(* Logix 5000 AddOnInstructionDefinition export AMCI_3601_AOP_Program_Blend_Move; software revision 20.03 *)

ADD_ON_INSTRUCTION AMCI_3601_AOP_Program_Blend_Move   (* revision 0.0 *)
// Revision note:
// 3/2020: Version 0 is the initial release
VAR_INPUT
   Status_Bits_MSW : INT; {required}
   Status_Bits_LSW : INT; {required}
        .9   // The 3601 module sets this bit to Acknowledge the receipt of a blend move programming block
   Number_of_Segments : INT; {required}
   Final_Move_Deceleration : INT; {required}
   Acceleration_Type_segments_9_to_16 : INT;
   Acceleration_Type_segments_1_to_8 : INT;
   Segment_1_Distance : DINT; {required}
   Segment_1_Programmed_Speed : DINT; {required}
   Segment_1_Acceleration_Deceleration : INT; {required}
   Segment_2_Distance : DINT; {required}
   Segment_2_Programmed_Speed : DINT; {required}
   Segment_2_Acceleration_Deceleration : INT; {required}
   Segment_3_Distance : DINT; {required}
   Segment_3_Programmed_Speed : DINT; {required}
   Segment_3_Acceleration_Deceleration : INT; {required}
   Segment_4_Distance : DINT; {required}
   Segment_4_Programmed_Speed : DINT; {required}
   Segment_4_Acceleration_Deceleration : INT; {required}
   Segment_5_Distance : DINT; {required}
   Segment_5_Programmed_Speed : DINT; {required}
   Segment_5_Acceleration_Deceleration : INT; {required}
   Segment_6_Distance : DINT; {required}
   Segment_6_Programmed_Speed : DINT; {required}
   Segment_6_Acceleration_Deceleration : INT; {required}
   Segment_7_Distance : DINT; {required}
   Segment_7_Programmed_Speed : DINT; {required}
   Segment_7_Acceleration_Deceleration : INT; {required}
   Segment_8_Distance : DINT; {required}
   Segment_8_Programmed_Speed : DINT; {required}
   Segment_8_Acceleration_Deceleration : INT; {required}
   Segment_9_Distance : DINT; {required}
   Segment_9_Programmed_Speed : DINT; {required}
   Segment_9_Acceleration_Deceleration : INT; {required}
   Segment_10_Distance : DINT; {required}
   Segment_10_Programmed_Speed : DINT; {required}
   Segment_10_Acceleration_Deceleration : INT; {required}
   Segment_11_Distance : DINT; {required}
   Segment_11_Programmed_Speed : DINT; {required}
   Segment_11_Acceleration_Deceleration : INT; {required}
   Segment_12_Distance : DINT; {required}
   Segment_12_Programmed_Speed : DINT; {required}
   Segment_12_Acceleration_Deceleration : INT; {required}
   Segment_13_Distance : DINT; {required}
   Segment_13_Programmed_Speed : DINT; {required}
   Segment_13_Acceleration_Deceleration : INT; {required}
   Segment_14_Distance : DINT; {required}
   Segment_14_Programmed_Speed : DINT; {required}
   Segment_14_Acceleration_Deceleration : INT; {required}
   Segment_15_Distance : DINT; {required}
   Segment_15_Programmed_Speed : DINT; {required}
   Segment_15_Acceleration_Deceleration : INT; {required}
   Segment_16_Distance : DINT; {required}
   Segment_16_Programmed_Speed : DINT; {required}
   Segment_16_Acceleration_Deceleration : INT; {required}
END_VAR
VAR_OUTPUT
   Blend_Move_Programmed : BOOL; {access Read Only, visible}
END_VAR
VAR_IN_OUT
   AMCI_3601_output_data : AM:1769_3601:O:0; {required}
END_VAR
VAR
   command_data_block : INT[8];
   Blend_Move_setup : INT[8] := ([1] := 768);
   Blend_Move_counter : COUNTER;
   Programmed_Speed : DINT;
   Distance : DINT;
   upper_result_X_1000 : DINT;
END_VAR

ROUTINE Logic   (* ladder *)
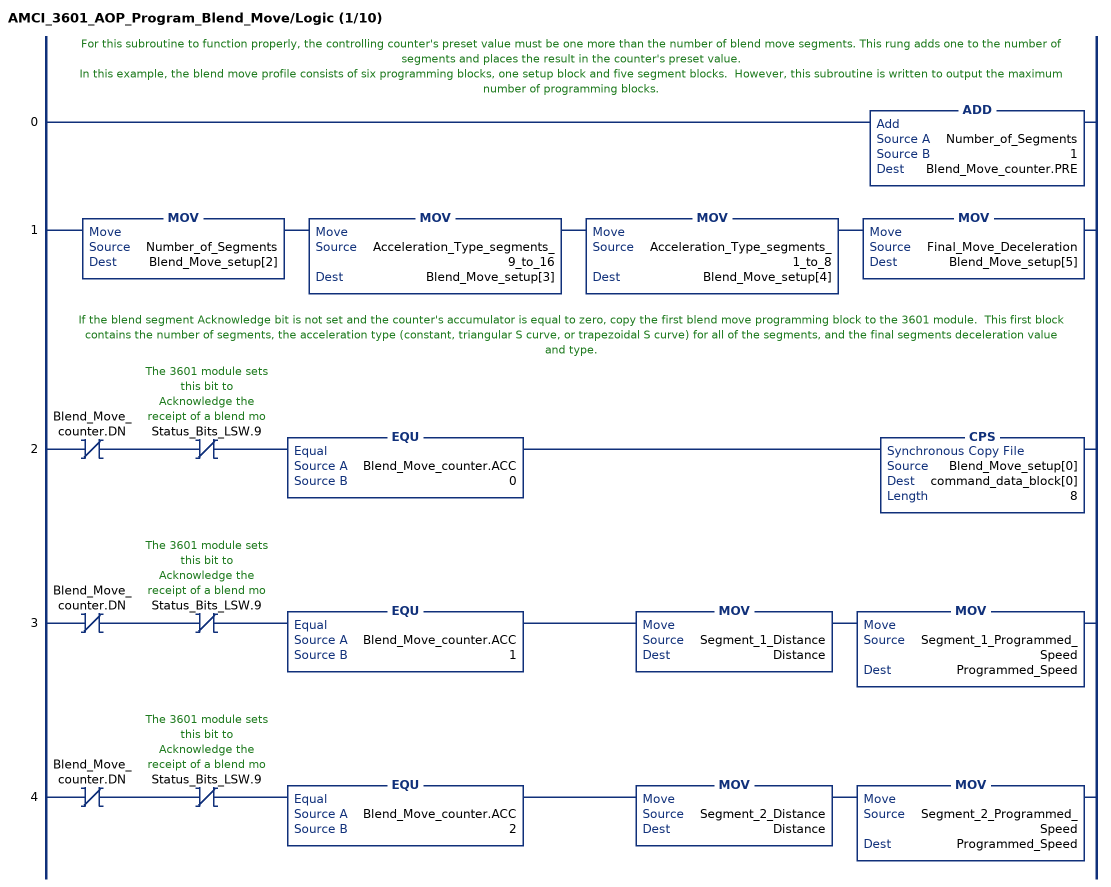
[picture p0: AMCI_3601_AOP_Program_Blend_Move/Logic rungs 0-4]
   // For this subroutine to function properly, the controlling counter's preset value must be one more than the number of blend move segments. This rung adds one to the number of segments and places the result in the counter's preset value.
   // In this example, the blend move profile consists of six programming blocks, one setup block and five segment blocks.  However, this subroutine is written to output the maximum number of programming blocks.
   0: ADD(Number_of_Segments,1,Blend_Move_counter.PRE);
   1: MOV(Number_of_Segments,Blend_Move_setup[2])MOV(Acceleration_Type_segments_9_to_16,Blend_Move_setup[3])MOV(Acceleration_Type_segments_1_to_8,Blend_Move_setup[4])MOV(Final_Move_Deceleration,Blend_Move_setup[5]);
   // If the blend segment Acknowledge bit is not set and the counter's accumulator is equal to zero, copy the first blend move programming block to the 3601 module.  This first block contains the number of segments, the acceleration type (constant, triangular S curve, or trapezoidal S curve) for all of the segments, and the final segments deceleration value and type.
   2: XIO(Blend_Move_counter.DN)XIO(Status_Bits_LSW.9)EQU(Blend_Move_counter.ACC,0)CPS(Blend_Move_setup[0],command_data_block[0],8);
   3: XIO(Blend_Move_counter.DN)XIO(Status_Bits_LSW.9)EQU(Blend_Move_counter.ACC,1)MOV(Segment_1_Distance,Distance)MOV(Segment_1_Programmed_Speed,Programmed_Speed);
   4: XIO(Blend_Move_counter.DN)XIO(Status_Bits_LSW.9)EQU(Blend_Move_counter.ACC,2)MOV(Segment_2_Distance,Distance)MOV(Segment_2_Programmed_Speed,Programmed_Speed);
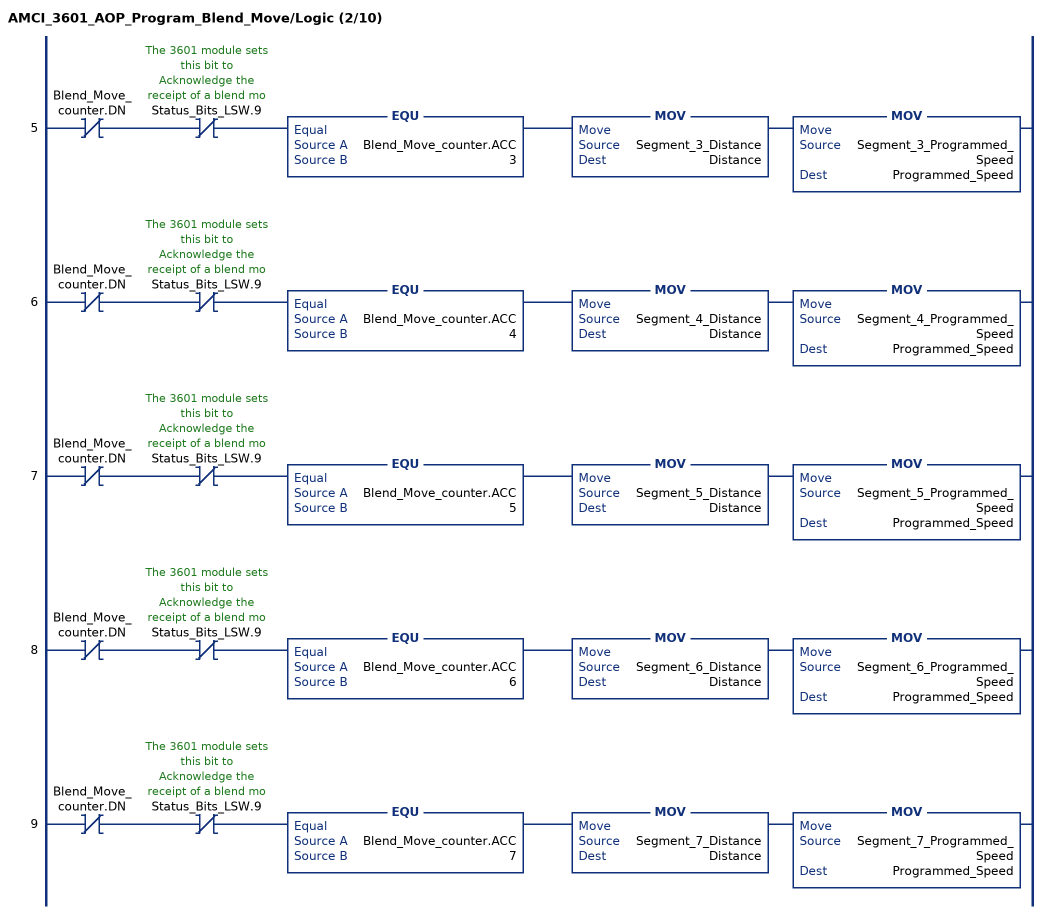
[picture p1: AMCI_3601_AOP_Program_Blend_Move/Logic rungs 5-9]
   5: XIO(Blend_Move_counter.DN)XIO(Status_Bits_LSW.9)EQU(Blend_Move_counter.ACC,3)MOV(Segment_3_Distance,Distance)MOV(Segment_3_Programmed_Speed,Programmed_Speed);
   6: XIO(Blend_Move_counter.DN)XIO(Status_Bits_LSW.9)EQU(Blend_Move_counter.ACC,4)MOV(Segment_4_Distance,Distance)MOV(Segment_4_Programmed_Speed,Programmed_Speed);
   7: XIO(Blend_Move_counter.DN)XIO(Status_Bits_LSW.9)EQU(Blend_Move_counter.ACC,5)MOV(Segment_5_Distance,Distance)MOV(Segment_5_Programmed_Speed,Programmed_Speed);
   8: XIO(Blend_Move_counter.DN)XIO(Status_Bits_LSW.9)EQU(Blend_Move_counter.ACC,6)MOV(Segment_6_Distance,Distance)MOV(Segment_6_Programmed_Speed,Programmed_Speed);
   9: XIO(Blend_Move_counter.DN)XIO(Status_Bits_LSW.9)EQU(Blend_Move_counter.ACC,7)MOV(Segment_7_Distance,Distance)MOV(Segment_7_Programmed_Speed,Programmed_Speed);
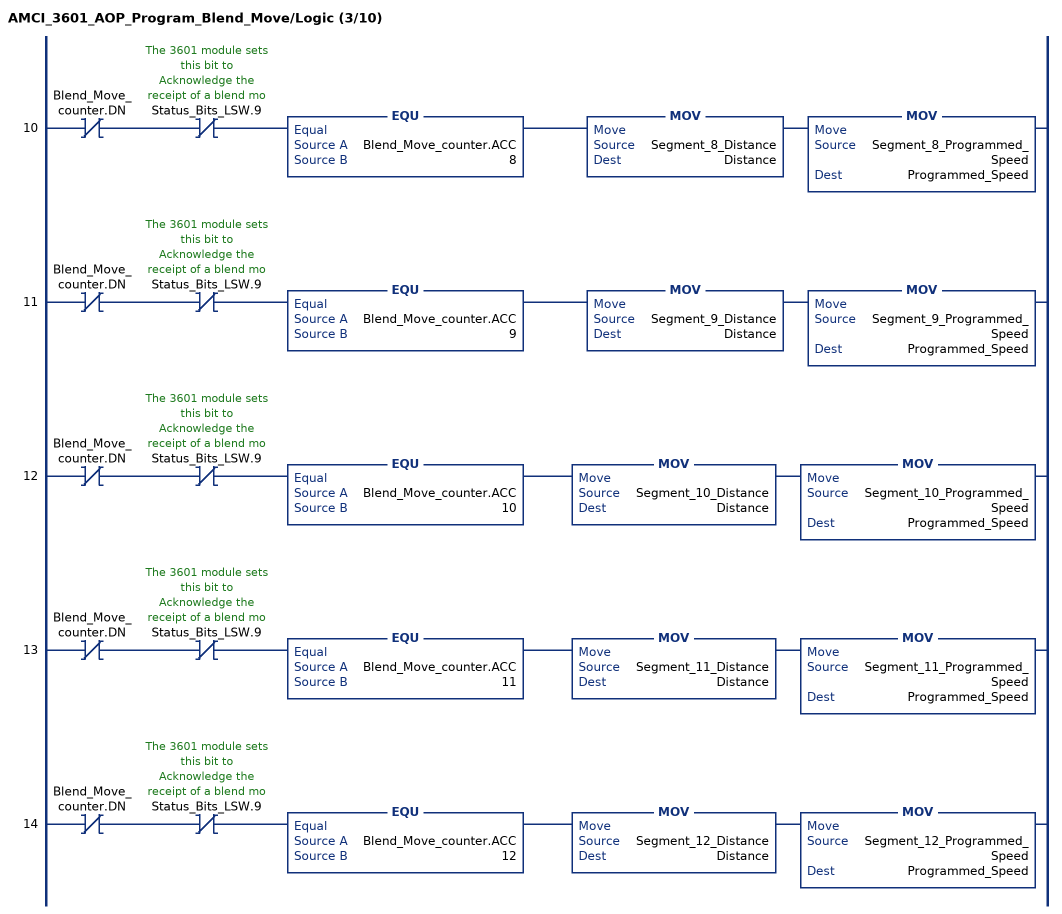
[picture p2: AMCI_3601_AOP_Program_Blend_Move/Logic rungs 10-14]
   10: XIO(Blend_Move_counter.DN)XIO(Status_Bits_LSW.9)EQU(Blend_Move_counter.ACC,8)MOV(Segment_8_Distance,Distance)MOV(Segment_8_Programmed_Speed,Programmed_Speed);
   11: XIO(Blend_Move_counter.DN)XIO(Status_Bits_LSW.9)EQU(Blend_Move_counter.ACC,9)MOV(Segment_9_Distance,Distance)MOV(Segment_9_Programmed_Speed,Programmed_Speed);
   12: XIO(Blend_Move_counter.DN)XIO(Status_Bits_LSW.9)EQU(Blend_Move_counter.ACC,10)MOV(Segment_10_Distance,Distance)MOV(Segment_10_Programmed_Speed,Programmed_Speed);
   13: XIO(Blend_Move_counter.DN)XIO(Status_Bits_LSW.9)EQU(Blend_Move_counter.ACC,11)MOV(Segment_11_Distance,Distance)MOV(Segment_11_Programmed_Speed,Programmed_Speed);
   14: XIO(Blend_Move_counter.DN)XIO(Status_Bits_LSW.9)EQU(Blend_Move_counter.ACC,12)MOV(Segment_12_Distance,Distance)MOV(Segment_12_Programmed_Speed,Programmed_Speed);
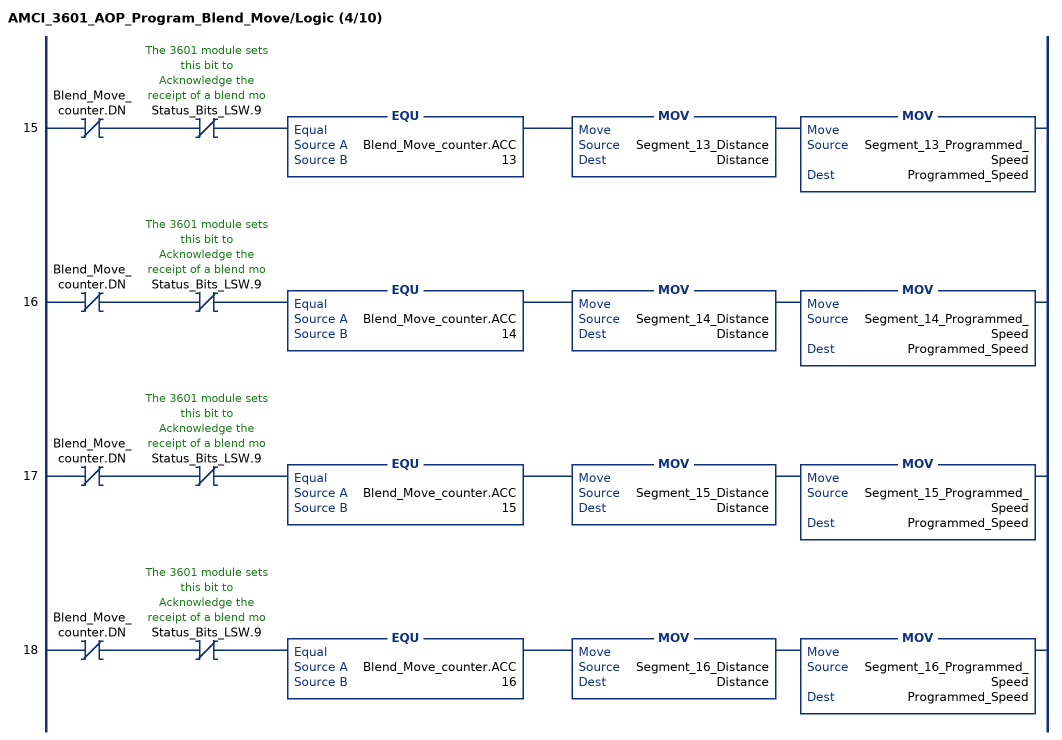
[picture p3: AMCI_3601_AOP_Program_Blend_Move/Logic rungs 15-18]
   15: XIO(Blend_Move_counter.DN)XIO(Status_Bits_LSW.9)EQU(Blend_Move_counter.ACC,13)MOV(Segment_13_Distance,Distance)MOV(Segment_13_Programmed_Speed,Programmed_Speed);
   16: XIO(Blend_Move_counter.DN)XIO(Status_Bits_LSW.9)EQU(Blend_Move_counter.ACC,14)MOV(Segment_14_Distance,Distance)MOV(Segment_14_Programmed_Speed,Programmed_Speed);
   17: XIO(Blend_Move_counter.DN)XIO(Status_Bits_LSW.9)EQU(Blend_Move_counter.ACC,15)MOV(Segment_15_Distance,Distance)MOV(Segment_15_Programmed_Speed,Programmed_Speed);
   18: XIO(Blend_Move_counter.DN)XIO(Status_Bits_LSW.9)EQU(Blend_Move_counter.ACC,16)MOV(Segment_16_Distance,Distance)MOV(Segment_16_Programmed_Speed,Programmed_Speed);
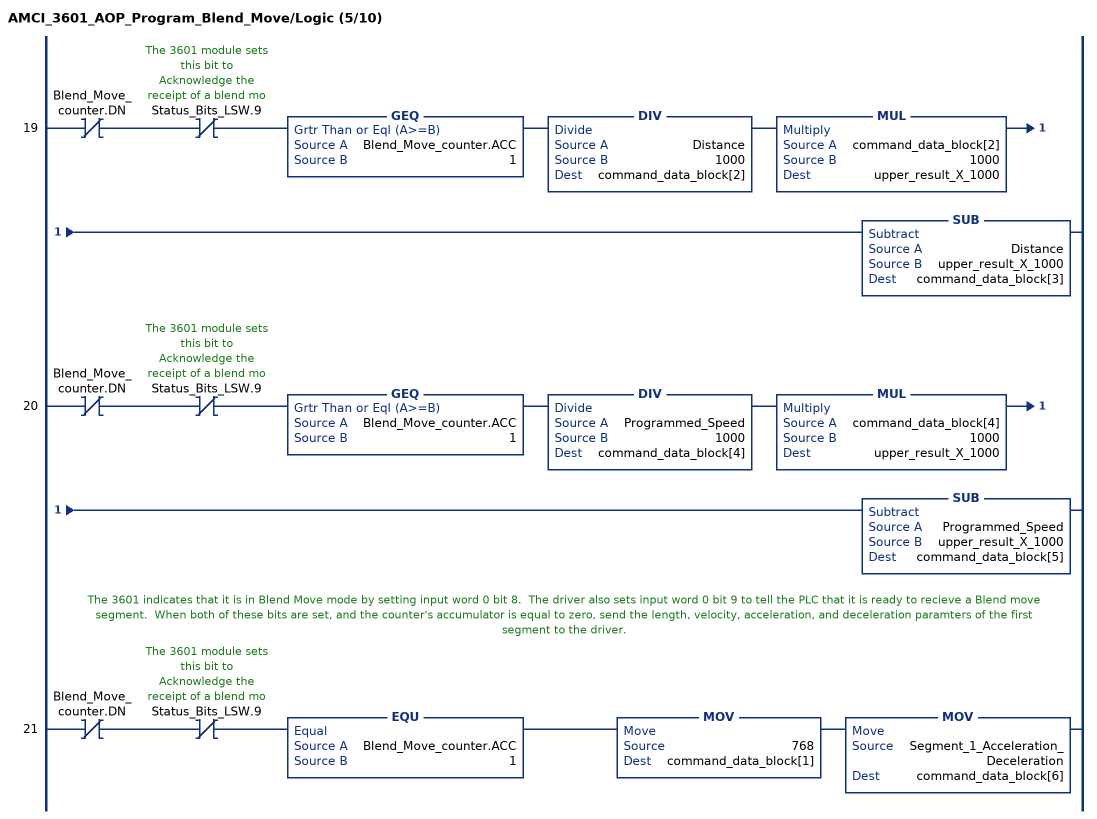
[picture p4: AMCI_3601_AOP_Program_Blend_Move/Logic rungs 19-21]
   19: XIO(Blend_Move_counter.DN)XIO(Status_Bits_LSW.9)GEQ(Blend_Move_counter.ACC,1)DIV(Distance,1000,command_data_block[2])MUL(command_data_block[2],1000,upper_result_X_1000)SUB(Distance,upper_result_X_1000,command_data_block[3]);
   20: XIO(Blend_Move_counter.DN)XIO(Status_Bits_LSW.9)GEQ(Blend_Move_counter.ACC,1)DIV(Programmed_Speed,1000,command_data_block[4])MUL(command_data_block[4],1000,upper_result_X_1000)SUB(Programmed_Speed,upper_result_X_1000,command_data_block[5]);
   // The 3601 indicates that it is in Blend Move mode by setting input word 0 bit 8.  The driver also sets input word 0 bit 9 to tell the PLC that it is ready to recieve a Blend move segment.  When both of these bits are set, and the counter's accumulator is equal to zero, send the length, velocity, acceleration, and deceleration paramters of the first segment to the driver.
   21: XIO(Blend_Move_counter.DN)XIO(Status_Bits_LSW.9)EQU(Blend_Move_counter.ACC,1)MOV(768,command_data_block[1])MOV(Segment_1_Acceleration_Deceleration,command_data_block[6]);
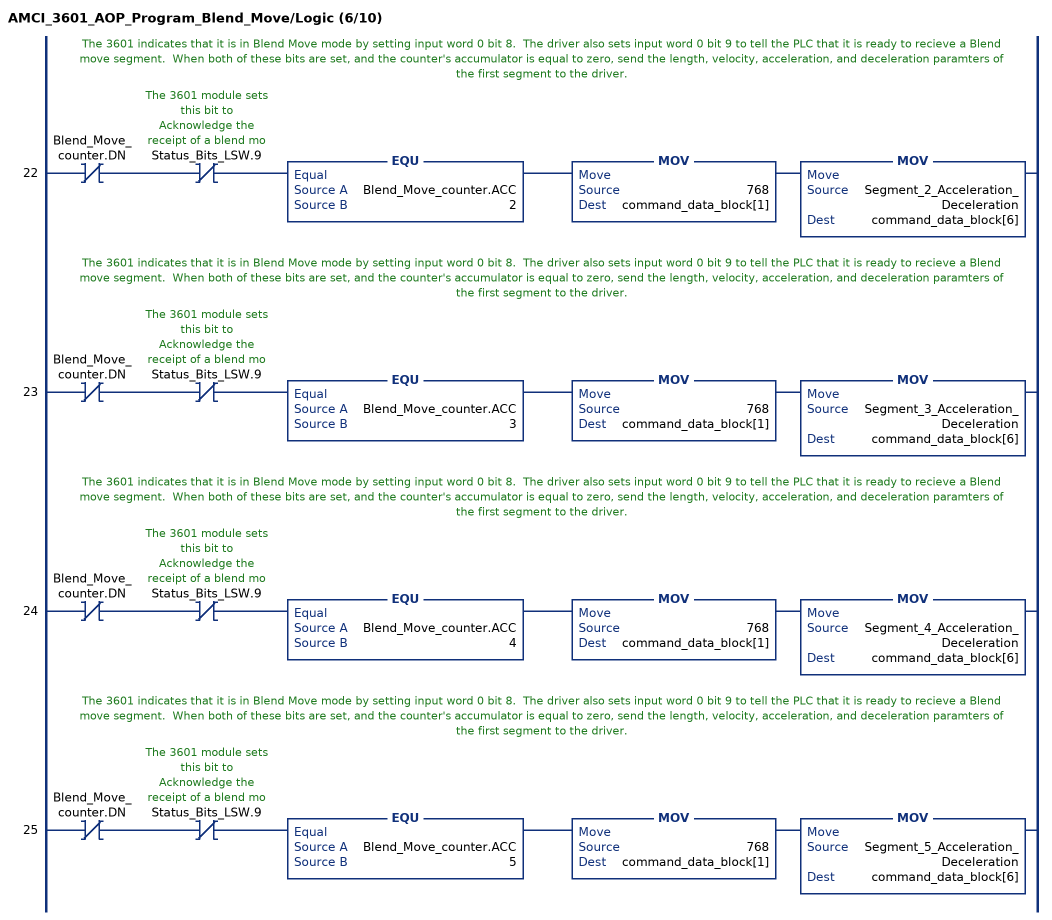
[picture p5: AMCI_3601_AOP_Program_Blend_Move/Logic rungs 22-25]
   // The 3601 indicates that it is in Blend Move mode by setting input word 0 bit 8.  The driver also sets input word 0 bit 9 to tell the PLC that it is ready to recieve a Blend move segment.  When both of these bits are set, and the counter's accumulator is equal to zero, send the length, velocity, acceleration, and deceleration paramters of the first segment to the driver.
   22: XIO(Blend_Move_counter.DN)XIO(Status_Bits_LSW.9)EQU(Blend_Move_counter.ACC,2)MOV(768,command_data_block[1])MOV(Segment_2_Acceleration_Deceleration,command_data_block[6]);
   // The 3601 indicates that it is in Blend Move mode by setting input word 0 bit 8.  The driver also sets input word 0 bit 9 to tell the PLC that it is ready to recieve a Blend move segment.  When both of these bits are set, and the counter's accumulator is equal to zero, send the length, velocity, acceleration, and deceleration paramters of the first segment to the driver.
   23: XIO(Blend_Move_counter.DN)XIO(Status_Bits_LSW.9)EQU(Blend_Move_counter.ACC,3)MOV(768,command_data_block[1])MOV(Segment_3_Acceleration_Deceleration,command_data_block[6]);
   // The 3601 indicates that it is in Blend Move mode by setting input word 0 bit 8.  The driver also sets input word 0 bit 9 to tell the PLC that it is ready to recieve a Blend move segment.  When both of these bits are set, and the counter's accumulator is equal to zero, send the length, velocity, acceleration, and deceleration paramters of the first segment to the driver.
   24: XIO(Blend_Move_counter.DN)XIO(Status_Bits_LSW.9)EQU(Blend_Move_counter.ACC,4)MOV(768,command_data_block[1])MOV(Segment_4_Acceleration_Deceleration,command_data_block[6]);
   // The 3601 indicates that it is in Blend Move mode by setting input word 0 bit 8.  The driver also sets input word 0 bit 9 to tell the PLC that it is ready to recieve a Blend move segment.  When both of these bits are set, and the counter's accumulator is equal to zero, send the length, velocity, acceleration, and deceleration paramters of the first segment to the driver.
   25: XIO(Blend_Move_counter.DN)XIO(Status_Bits_LSW.9)EQU(Blend_Move_counter.ACC,5)MOV(768,command_data_block[1])MOV(Segment_5_Acceleration_Deceleration,command_data_block[6]);
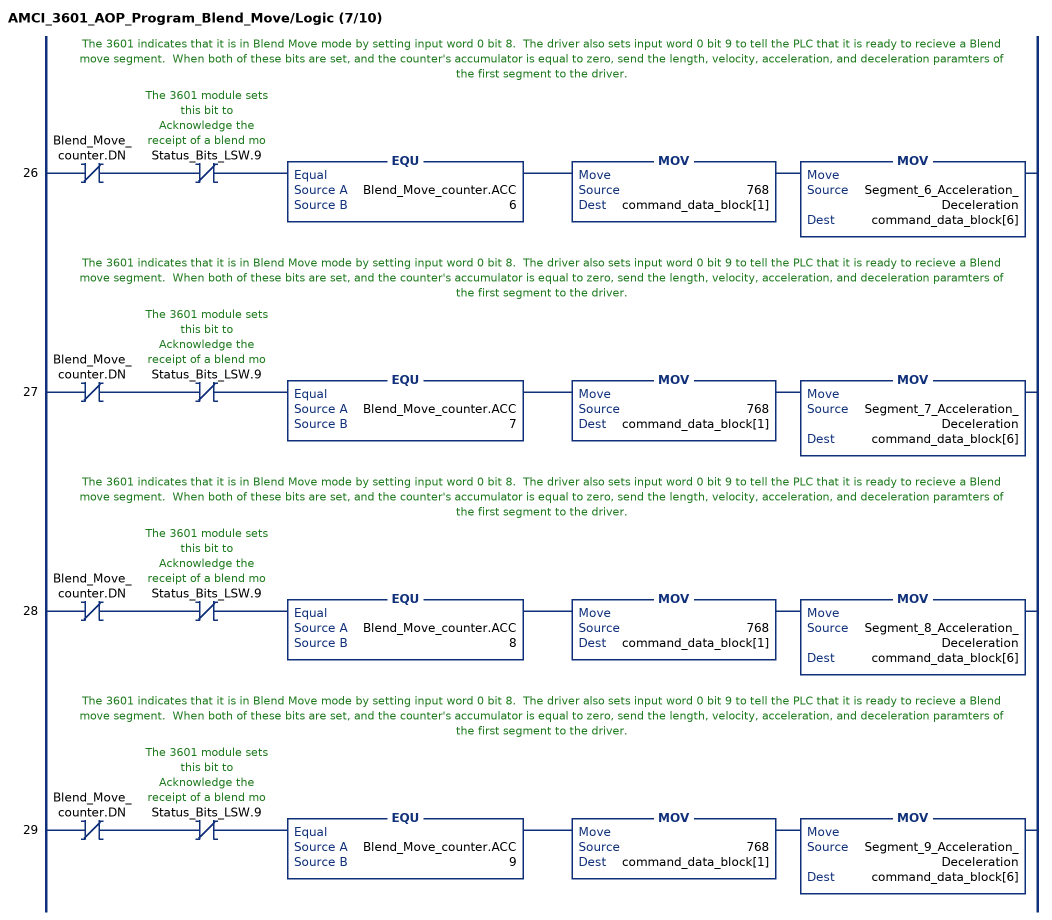
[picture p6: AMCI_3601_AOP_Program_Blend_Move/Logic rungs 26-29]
   // The 3601 indicates that it is in Blend Move mode by setting input word 0 bit 8.  The driver also sets input word 0 bit 9 to tell the PLC that it is ready to recieve a Blend move segment.  When both of these bits are set, and the counter's accumulator is equal to zero, send the length, velocity, acceleration, and deceleration paramters of the first segment to the driver.
   26: XIO(Blend_Move_counter.DN)XIO(Status_Bits_LSW.9)EQU(Blend_Move_counter.ACC,6)MOV(768,command_data_block[1])MOV(Segment_6_Acceleration_Deceleration,command_data_block[6]);
   // The 3601 indicates that it is in Blend Move mode by setting input word 0 bit 8.  The driver also sets input word 0 bit 9 to tell the PLC that it is ready to recieve a Blend move segment.  When both of these bits are set, and the counter's accumulator is equal to zero, send the length, velocity, acceleration, and deceleration paramters of the first segment to the driver.
   27: XIO(Blend_Move_counter.DN)XIO(Status_Bits_LSW.9)EQU(Blend_Move_counter.ACC,7)MOV(768,command_data_block[1])MOV(Segment_7_Acceleration_Deceleration,command_data_block[6]);
   // The 3601 indicates that it is in Blend Move mode by setting input word 0 bit 8.  The driver also sets input word 0 bit 9 to tell the PLC that it is ready to recieve a Blend move segment.  When both of these bits are set, and the counter's accumulator is equal to zero, send the length, velocity, acceleration, and deceleration paramters of the first segment to the driver.
   28: XIO(Blend_Move_counter.DN)XIO(Status_Bits_LSW.9)EQU(Blend_Move_counter.ACC,8)MOV(768,command_data_block[1])MOV(Segment_8_Acceleration_Deceleration,command_data_block[6]);
   // The 3601 indicates that it is in Blend Move mode by setting input word 0 bit 8.  The driver also sets input word 0 bit 9 to tell the PLC that it is ready to recieve a Blend move segment.  When both of these bits are set, and the counter's accumulator is equal to zero, send the length, velocity, acceleration, and deceleration paramters of the first segment to the driver.
   29: XIO(Blend_Move_counter.DN)XIO(Status_Bits_LSW.9)EQU(Blend_Move_counter.ACC,9)MOV(768,command_data_block[1])MOV(Segment_9_Acceleration_Deceleration,command_data_block[6]);
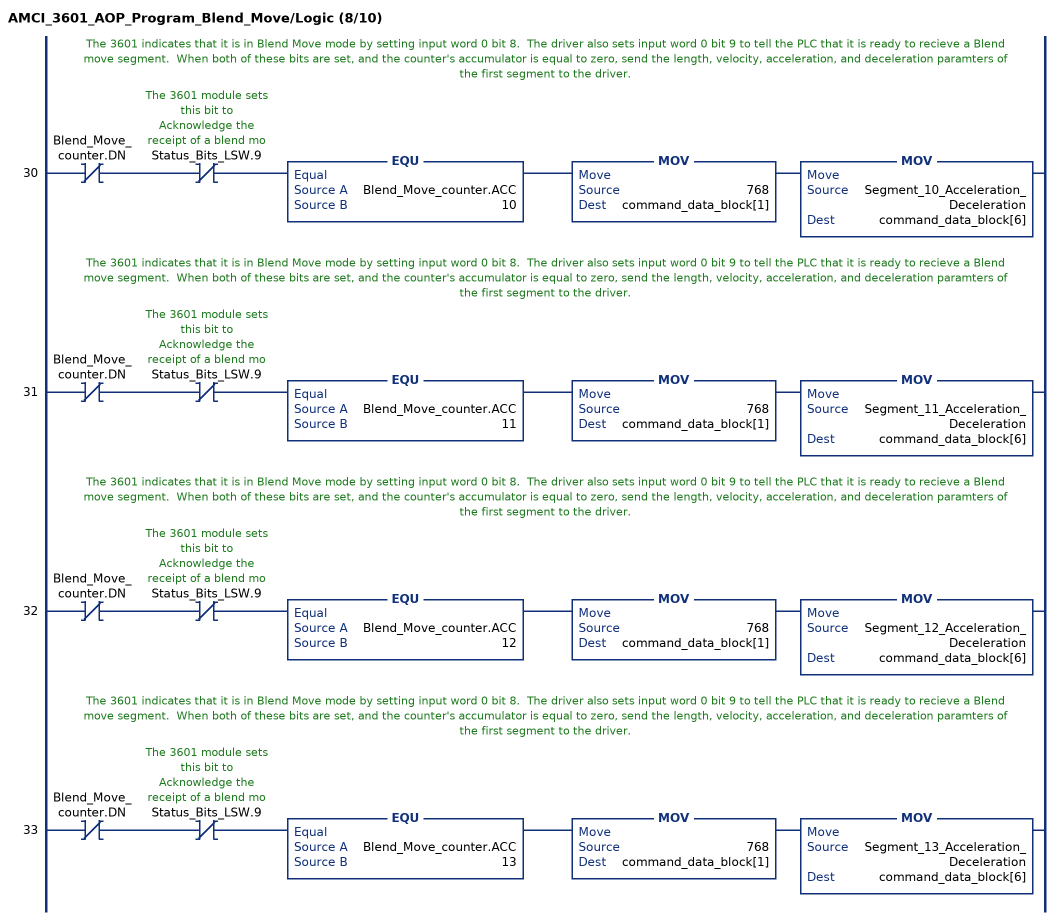
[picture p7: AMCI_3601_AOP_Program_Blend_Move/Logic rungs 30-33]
   // The 3601 indicates that it is in Blend Move mode by setting input word 0 bit 8.  The driver also sets input word 0 bit 9 to tell the PLC that it is ready to recieve a Blend move segment.  When both of these bits are set, and the counter's accumulator is equal to zero, send the length, velocity, acceleration, and deceleration paramters of the first segment to the driver.
   30: XIO(Blend_Move_counter.DN)XIO(Status_Bits_LSW.9)EQU(Blend_Move_counter.ACC,10)MOV(768,command_data_block[1])MOV(Segment_10_Acceleration_Deceleration,command_data_block[6]);
   // The 3601 indicates that it is in Blend Move mode by setting input word 0 bit 8.  The driver also sets input word 0 bit 9 to tell the PLC that it is ready to recieve a Blend move segment.  When both of these bits are set, and the counter's accumulator is equal to zero, send the length, velocity, acceleration, and deceleration paramters of the first segment to the driver.
   31: XIO(Blend_Move_counter.DN)XIO(Status_Bits_LSW.9)EQU(Blend_Move_counter.ACC,11)MOV(768,command_data_block[1])MOV(Segment_11_Acceleration_Deceleration,command_data_block[6]);
   // The 3601 indicates that it is in Blend Move mode by setting input word 0 bit 8.  The driver also sets input word 0 bit 9 to tell the PLC that it is ready to recieve a Blend move segment.  When both of these bits are set, and the counter's accumulator is equal to zero, send the length, velocity, acceleration, and deceleration paramters of the first segment to the driver.
   32: XIO(Blend_Move_counter.DN)XIO(Status_Bits_LSW.9)EQU(Blend_Move_counter.ACC,12)MOV(768,command_data_block[1])MOV(Segment_12_Acceleration_Deceleration,command_data_block[6]);
   // The 3601 indicates that it is in Blend Move mode by setting input word 0 bit 8.  The driver also sets input word 0 bit 9 to tell the PLC that it is ready to recieve a Blend move segment.  When both of these bits are set, and the counter's accumulator is equal to zero, send the length, velocity, acceleration, and deceleration paramters of the first segment to the driver.
   33: XIO(Blend_Move_counter.DN)XIO(Status_Bits_LSW.9)EQU(Blend_Move_counter.ACC,13)MOV(768,command_data_block[1])MOV(Segment_13_Acceleration_Deceleration,command_data_block[6]);
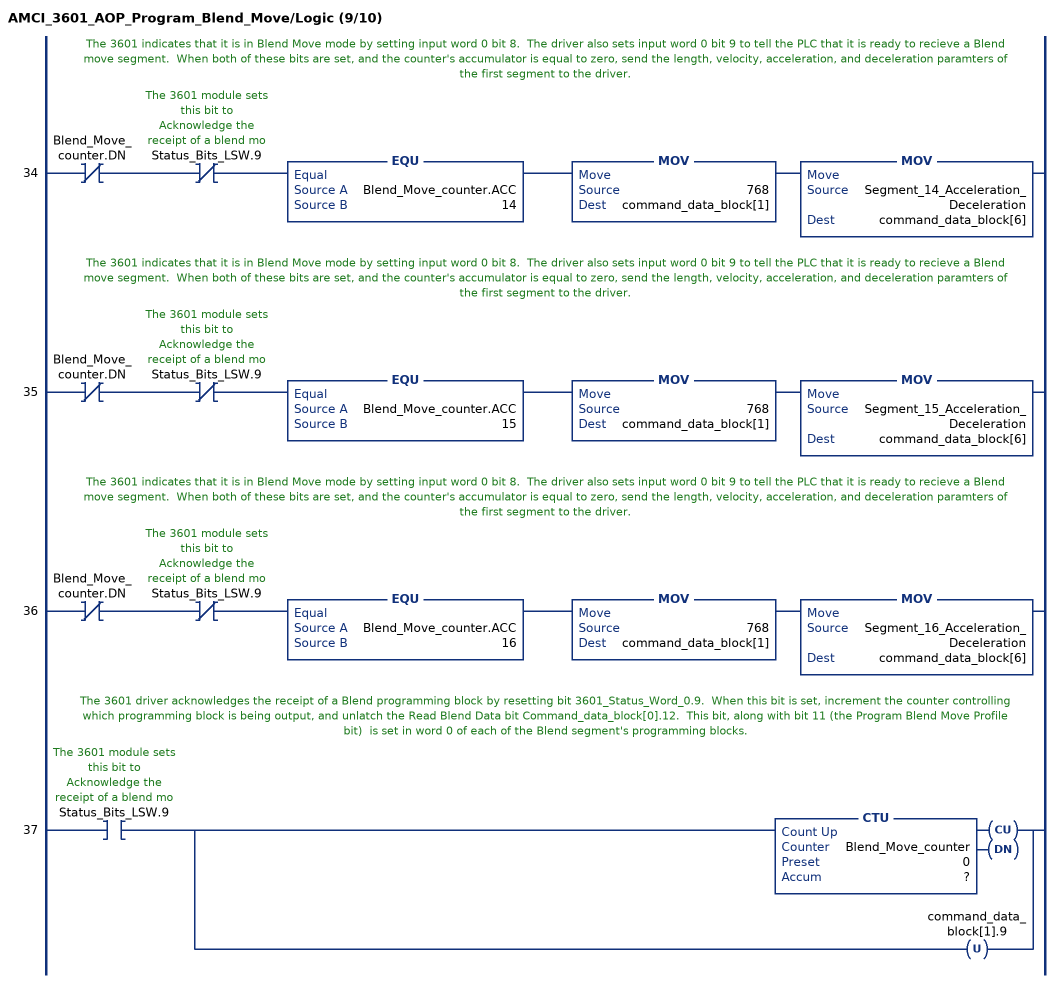
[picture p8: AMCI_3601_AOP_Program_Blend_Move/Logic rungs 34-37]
   // The 3601 indicates that it is in Blend Move mode by setting input word 0 bit 8.  The driver also sets input word 0 bit 9 to tell the PLC that it is ready to recieve a Blend move segment.  When both of these bits are set, and the counter's accumulator is equal to zero, send the length, velocity, acceleration, and deceleration paramters of the first segment to the driver.
   34: XIO(Blend_Move_counter.DN)XIO(Status_Bits_LSW.9)EQU(Blend_Move_counter.ACC,14)MOV(768,command_data_block[1])MOV(Segment_14_Acceleration_Deceleration,command_data_block[6]);
   // The 3601 indicates that it is in Blend Move mode by setting input word 0 bit 8.  The driver also sets input word 0 bit 9 to tell the PLC that it is ready to recieve a Blend move segment.  When both of these bits are set, and the counter's accumulator is equal to zero, send the length, velocity, acceleration, and deceleration paramters of the first segment to the driver.
   35: XIO(Blend_Move_counter.DN)XIO(Status_Bits_LSW.9)EQU(Blend_Move_counter.ACC,15)MOV(768,command_data_block[1])MOV(Segment_15_Acceleration_Deceleration,command_data_block[6]);
   // The 3601 indicates that it is in Blend Move mode by setting input word 0 bit 8.  The driver also sets input word 0 bit 9 to tell the PLC that it is ready to recieve a Blend move segment.  When both of these bits are set, and the counter's accumulator is equal to zero, send the length, velocity, acceleration, and deceleration paramters of the first segment to the driver.
   36: XIO(Blend_Move_counter.DN)XIO(Status_Bits_LSW.9)EQU(Blend_Move_counter.ACC,16)MOV(768,command_data_block[1])MOV(Segment_16_Acceleration_Deceleration,command_data_block[6]);
   // The 3601 driver acknowledges the receipt of a Blend programming block by resetting bit 3601_Status_Word_0.9.  When this bit is set, increment the counter controlling which programming block is being output, and unlatch the Read Blend Data bit Command_data_block[0].12.  This bit, along with bit 11 (the Program Blend Move Profile bit)  is set in word 0 of each of the Blend segment's programming blocks.
   37: XIC(Status_Bits_LSW.9)[CTU(Blend_Move_counter,?,?) ,OTU(command_data_block[1].9) ];
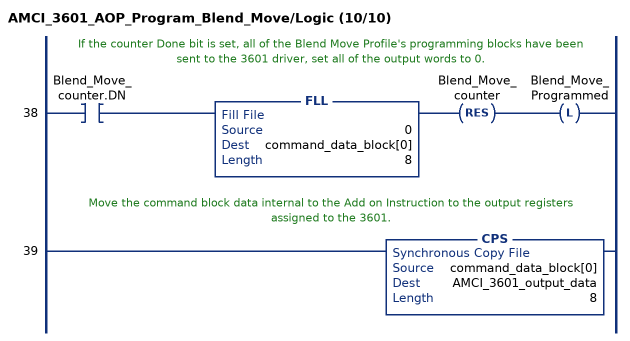
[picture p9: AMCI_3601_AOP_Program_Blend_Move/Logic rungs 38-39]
   // If the counter Done bit is set, all of the Blend Move Profile's programming blocks have been sent to the 3601 driver, set all of the output words to 0.
   38: XIC(Blend_Move_counter.DN)FLL(0,command_data_block[0],8)RES(Blend_Move_counter)OTL(Blend_Move_Programmed);
   // Move the command block data internal to the Add on Instruction to the output registers assigned to the 3601.
   39: CPS(command_data_block[0],AMCI_3601_output_data,8);
END_ROUTINE
END_ADD_ON_INSTRUCTION
